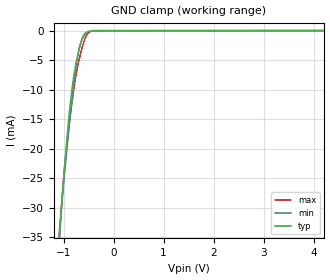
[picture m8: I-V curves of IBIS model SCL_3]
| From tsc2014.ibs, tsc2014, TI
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|   3.0V SCL Model
[Model] SCL_3
Model_type Input
Vinl = 0.9
Vinh = 2.1
|   typ   min   max
C_comp   2.7972710e-12   2.6509420e-12   2.9513260e-12
|Where nom PVT is NOM Process, 3V,27C
|   Fast PVT is Strong Process, 3.45V, -40C
|   Slow PVT is Weak Process, 2.65V, 85C
[Model Spec]
Vinl   0.9   0.795   1.035
Vinh   2.1   1.855   2.415
| VINL 0.3 DVDD, VINH 0.7 DVDD
[Voltage Range]   3   2.65   3.45
[Temperature Range]   27   85   -40
[Power Clamp Reference]   3   2.65   3.45
[GND Clamp Reference]   0   0   0
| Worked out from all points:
|   GND clamp passes 1 mA (typ) near -0.60 V on its own axis
[GND Clamp]
|   Voltage   I(typ)   I(min)   I(max)
-3V       -288mA     -228.6mA   -402.1mA
-1.088V   -35.53mA   -34.31mA   -36.22mA
-1.071V   -33.47mA   -32.69mA   -33.78mA
-1.003V   -25.75mA   -26.45mA   -25.41mA
-945.3mV  -19.58mA   -21.22mA   -20.21mA
-879.3mV  -13.49mA   -15.59mA   -15.35mA
-797.3mV  -7.828mA   -9.255mA   -10.04mA
-689.8mV  -3.118mA   -3.175mA   -4.977mA
-623.1mV  -1.37mA    -1.231mA   -2.736mA
-553.3mV  -455.2uA   -323.8uA   -1.027mA
-419.9mV  -16.89uA   -19.58uA   -28.78uA
6V        0A         0A         0A
[POWER Clamp]
|   SCR cell used for ESD function. Effects occurr above VDD x 2
|   Voltage   I(typ)   I(min)   I(max)
-3V       0A         0A         0A
0V        0A         0A         0A
6V        0A         0A         0A
